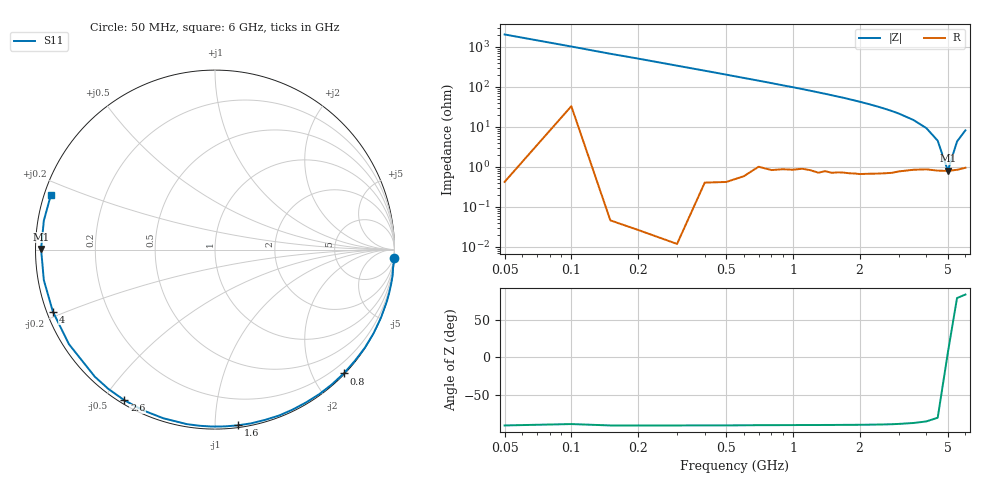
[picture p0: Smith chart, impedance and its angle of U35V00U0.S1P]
! SIEMENS Discrete & RF Semiconductors
! BBY53-02W
! Si Tuning Diode in SCD-80
! VR = 5 V
! S-Parameters:  September  1997
# GHz  S  MA  R  50
!  f  S11
! GHz  MAG  ANG
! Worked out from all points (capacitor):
!   34 points, 50 MHz to 6 GHz, reference 50 ohm
!   read as one part to ground: C = 1.56 pF near 50 MHz
!   lowest |Z| = 792 mohm at 5 GHz (marker M1)
!   series resonance near 4.99 GHz, so ESL is about 650 pH
!   S11 on the Smith chart (normalised r, x): 50 MHz: 0, -41; 800 MHz: 0.02, -2.48; 1.6 GHz: 0.01, -1.14; 2.6 GHz: 0.01, -0.57; 4 GHz: 0.02, -0.18; 6 GHz: 0.02, +0.16
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0.05  1 -2.8
0.2  1 -11.2
0.3  1 -16.8
0.4  0.9994 -22.3
0.5  0.999 -27.8
0.6  0.9981 -33.3
0.8  0.9954 -43.9
0.9  0.994 -49.2
1  0.9931 -54.1
1.1  0.9913 -59.1
1.2  0.9908 -64.1
1.3  0.9909 -68.9
1.4  0.9889 -73.6
1.5  0.9888 -78.2
1.6  0.9875 -82.6
1.8  0.9861 -91.2
2  0.9848 -99.3
2.2  0.9829 -107.0
2.4  0.9812 -114.2
2.6  0.9794 -121.0
2.8  0.9776 -127.4
3  0.9745 -133.4
3.5  0.9695 -147.1
4  0.9672 -159.1
4.5  0.9687 -169.9
5  0.969 179.8
5.5  0.9672 170.4
6  0.9638 161.6
